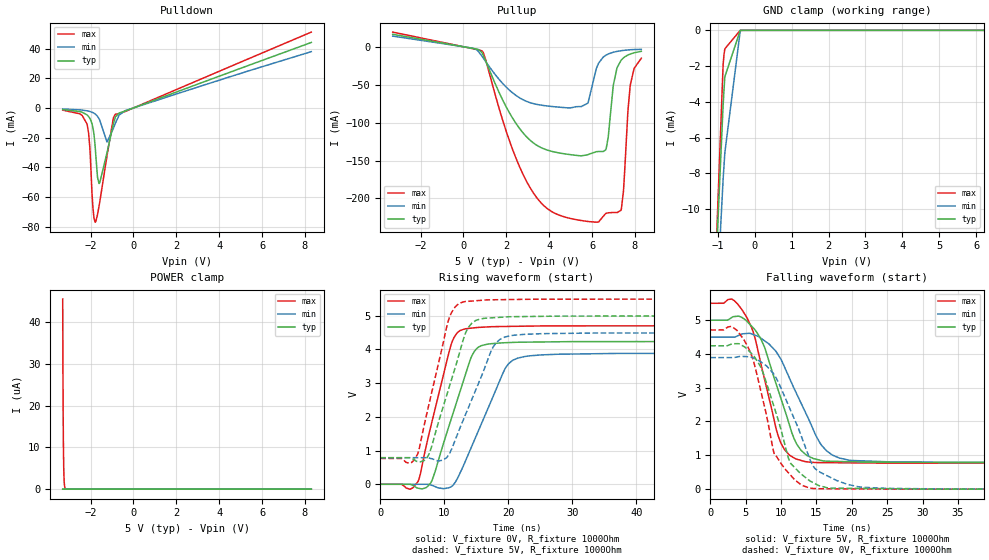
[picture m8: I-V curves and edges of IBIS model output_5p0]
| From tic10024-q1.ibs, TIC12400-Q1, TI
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|   output_5p0 Model
[Model]   output_5p0
Model_type   3-state
Polarity   Non-Inverting
Vmeas = 2.5
Vref = 0
Cref = 2pF
Rref = 100000
|   typ   min   max
C_comp   1.89513E-12F   1.76865E-12F   1.96627E-12F
| Where nom  PVT is Nominal Process, 5.0V, 27C
|   Fast PVT is Strong Process,  5.5V, -40C
|   Slow PVT is Weak Process,   4.5V, 150C
[Voltage Range]   5   4.5   5.5
|Junction Temperature
[Temperature Range]   27   150   -40
[Pullup Reference]   5   4.5   5.5
[Pulldown Reference]   0   0   0
[Power Clamp Reference]   5   4.5   5.5
[GND Clamp Reference]   0   0   0
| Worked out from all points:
|   slope of the pulldown table from 0 to 0.75 V, typ, clamps not added: 187 ohm
|   slope of the pullup table from 0 to 0.75 V, typ, clamps not added: 153 ohm
|   falling waveform, V_fixture 5V, R_fixture 1000Ohm: 20-80 % time 3.86ns typ, 4.88ns min, 3.2ns max; typ from 4.99 V to 0.787 V
|   rising waveform, V_fixture 0V, R_fixture 1000Ohm: 20-80 % time 4.24ns typ, 5.24ns min, 3.58ns max; typ from 0 V to 4.24 V
|   rising waveform, V_fixture 5V, R_fixture 1000Ohm: 20-80 % time 3.98ns typ, 4.75ns min, 3.41ns max; typ from 0.787 V to 4.99 V
|   falling waveform, V_fixture 0V, R_fixture 1000Ohm: 20-80 % time 3.63ns typ, 4.57ns min, 3.31ns max; typ from 4.24 V to 0 V
[Pulldown]
|   Voltage   I(typ)   I(min)   I(max)
-3.3V     -1.097mA   -695.2uA   -1.466mA
-2.175V   -4.562mA   -1.892mA   -10.52mA
-2.036V   -6.947mA   -2.362mA   -26.3mA
-1.885V   -13.7mA    -3.179mA   -67.98mA
-1.78V    -26.97mA   -4.105mA   -76.83mA
-1.676V   -46.66mA   -5.611mA   -71.69mA
-1.572V   -50.28mA   -8.233mA   -63.26mA
-1.235V   -30.24mA   -22.86mA   -32.37mA
-933.6mV  -10.71mA   -13.6mA    -6.584mA
-840.8mV  -5.943mA   -10.21mA   -4.197mA
-388.4mV  -2.082mA   -1.836mA   -2.4mA
8.3V      44.07mA    37.89mA    51.04mA
[GND Clamp]
|   Voltage   I(typ)   I(min)   I(max)
-3.3V     -1.398A    -1.627A    -1.283A
-1.224V   -21.32mA   -23.14mA   -22.27mA
-852.4mV  -4.187mA   -8.335mA   -1.912mA
-829.2mV  -3.361mA   -7.588mA   -1.372mA
-806mV    -2.599mA   -6.852mA   -1.034mA
-388.4mV  -167nA     -14.94uA   -102.3nA
8.3V      0A         0A         0A
[Pullup]
|   Voltage   I(typ)   I(min)   I(max)
-3.3V     16.46mA    14.08mA    19.37mA
852.8mV   -7.181mA   -12mA      -5.214mA
2.152V    -87.32mA   -57.36mA   -124.3mA
3.126V    -123.6mA   -73.83mA   -186.6mA
5.818V    -142.1mA   -73.64mA   -230.4mA
6.2V      -138.3mA   -28.73mA   -231.3mA
6.664V    -133.8mA   -10.81mA   -219.6mA
6.989V    -51.23mA   -7.225mA   -218.5mA
7.349V    -18.1mA    -5.233mA   -215.7mA
7.465V    -14.66mA   -4.799mA   -190.8mA
7.778V    -9.578mA   -3.916mA   -52.25mA
8.3V      -6.001mA   -3.377mA   -15.06mA
[POWER Clamp]
|   Voltage   I(typ)   I(min)   I(max)
-3.3V     441.6pA    1.98nA     45.52uA
-3.288V   220.8pA    990pA      27.83uA
-3.277V   0A         0A         16.55uA
-3.265V   0A         0A         9.625uA
-3.254V   0A         0A         5.513uA
-3.242V   0A         0A         3.123uA
-3.23V    0A         0A         1.754uA
-3.219V   0A         0A         976.7nA
-3.207V   0A         0A         537.3nA
-3.172V   0A         0A         72.16nA
8.3V      0A         0A         0A
[Ramp]
R_load = 1000
|   typ   min   max
dV/dt_r   2.542/4.23943e-09   2.33278/5.24097e-09   2.8218/3.58567e-09
dV/dt_f   2.52315/3.85021e-09   2.22167/4.86052e-09   2.83549/3.18732e-09
[Falling Waveform]
V_fixture = 5V
V_fixture_min = 4.5V
V_fixture_max = 5.5V
R_fixture = 1000Ohm
C_fixture = 0F
|   Time   V(typ)   V(min)   V(max)
0s        4.992V     4.491V     5.492V
3.404ns   5.1V       4.491V     5.569V
5.229ns   4.949V     4.601V     5.045V
6.571ns   4.636V     4.53V      4.249V
9.858ns   2.759V     3.883V     1.426V
11.82ns   1.507V     2.989V     926.5mV
13.33ns   1.052V     2.321V     818.4mV
16.44ns   826.9mV    1.133V     783.4mV
19.88ns   810.5mV    848.9mV    777.7mV
100ns     786.5mV    787.9mV    766.1mV
[Rising Waveform]
V_fixture = 0V
V_fixture_min = 0V
V_fixture_max = 0V
R_fixture = 1000Ohm
C_fixture = 0F
|   Time   V(typ)   V(min)   V(max)
0s        -52.84uV   31.26uV    -36.39uV
4.647ns   -183.3uV   -122.1uV   -145.5mV
5.883ns   -115.8mV   -162.9uV   76.92mV
8.01ns    86.98mV    -29.39mV   1.807V
10.99ns   1.881V     -80.74mV   4.094V
13.15ns   3.163V     620.8mV    4.604V
15.33ns   4.067V     1.591V     4.651V
19.64ns   4.198V     3.476V     4.68V
22.42ns   4.213V     3.783V     4.687V
100ns     4.237V     3.888V     4.703V
[Rising Waveform]
V_fixture = 5V
V_fixture_min = 4.5V
V_fixture_max = 5.5V
R_fixture = 1000Ohm
C_fixture = 0F
|   Time   V(typ)   V(min)   V(max)
0s        786.5mV    787.9mV    766.1mV
4.596ns   786.4mV    788mV      623.7mV
5.784ns   675.6mV    788mV      878.7mV
7.613ns   896.3mV    778mV      2.38V
10.6ns    2.785V     847.3mV    4.836V
12.92ns   4.269V     1.889V     5.406V
14.38ns   4.793V     2.556V     5.435V
17.55ns   4.937V     4.046V     5.471V
20.35ns   4.968V     4.406V     5.478V
100ns     4.992V     4.491V     5.492V
[Falling Waveform]
|Gnd
V_fixture = 0V
V_fixture_min = 0V
V_fixture_max = 0V
R_fixture = 1000Ohm
C_fixture = 0F
|   Time   V(typ)   V(min)   V(max)
0s        4.237V     3.888V     4.703V
3.763ns   4.298V     3.905V     4.695V
5.282ns   4.121V     3.913V     4.218V
6.363ns   3.875V     3.853V     3.591V
9.043ns   2.415V     3.378V     1.035V
11.31ns   780.6mV    2.348V     421.3mV
13.99ns   256.8mV    934.7mV    35.73mV
15.55ns   94.14mV    497.6mV    12.42mV
21.46ns   22.04mV    56.57mV    6.81mV
100ns     -52.84uV   31.26uV    -36.39uV
